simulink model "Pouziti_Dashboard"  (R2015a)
settings: Solver=ode45  StartTime=0.0  StopTime=inf  MaxStep=0.001  RelTol=1e-3
PreLoadFcn:
  | A1 = 0.2;
  | A01 = 0.001;
  | 
  | A2 = 0.2;
  | A02 = 0.001;
  | 
  | g = 9.81;

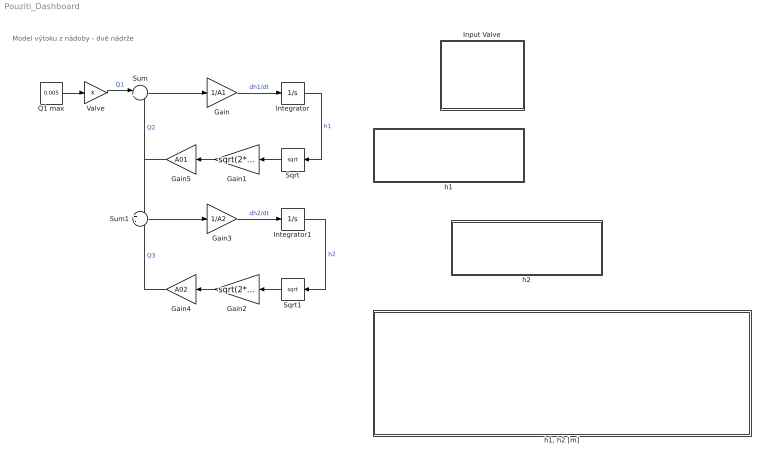
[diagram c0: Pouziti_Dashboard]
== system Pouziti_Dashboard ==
  note: Model výtoku z nádoby - dvě nádrže
  Gain : Gain  Gain=1/A1
  Gain1 : Gain  Gain=sqrt(2*g)
  Gain2 : Gain  Gain=sqrt(2*g)
  Gain3 : Gain  Gain=1/A2
  Gain4 : Gain  Gain=A02
  Gain5 : Gain  Gain=A01
  Input Valve : Subsystem  DialogController=hmiCreateDDGDialog  IsWebBlock=on
  Integrator : Integrator  LimitOutput=on  LowerSaturationLimit=0
  Integrator1 : Integrator  LimitOutput=on  LowerSaturationLimit=0
  Q1 max : Constant  Value=0.005
  Sqrt : Sqrt
  Sqrt1 : Sqrt
  Sum : Sum  Inputs=|+-
  Sum1 : Sum  Inputs=+-
  Valve : Gain
  h1 : Subsystem  DialogController=hmiCreateDDGDialog  IsWebBlock=on
  "h1, h2 [m]" : Subsystem  DialogController=hmiCreateDDGDialog  IsWebBlock=on
  h2 : Subsystem  DialogController=hmiCreateDDGDialog  IsWebBlock=on
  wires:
  Gain/1 -> Integrator/1  "dh1/dt"
  Q1 max/1 -> Valve/1
  Integrator/1 -> Sqrt/1  "h1"
  Sqrt/1 -> Gain1/1
  Gain1/1 -> Gain5/1
  Sum1/1 -> Gain3/1
  Integrator1/1 -> Sqrt1/1  "h2"
  Sqrt1/1 -> Gain2/1
  Gain4/1 -> Sum1/2  "Q3"
  Sum/1 -> Gain/1
  Gain3/1 -> Integrator1/1  "dh2/dt"
  Gain2/1 -> Gain4/1
  Gain5/1 -> Sum1/1, Sum/2  "Q2"
  Valve/1 -> Sum/1  "Q1"

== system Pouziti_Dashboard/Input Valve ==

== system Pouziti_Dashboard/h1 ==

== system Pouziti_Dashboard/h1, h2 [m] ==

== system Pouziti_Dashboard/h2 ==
